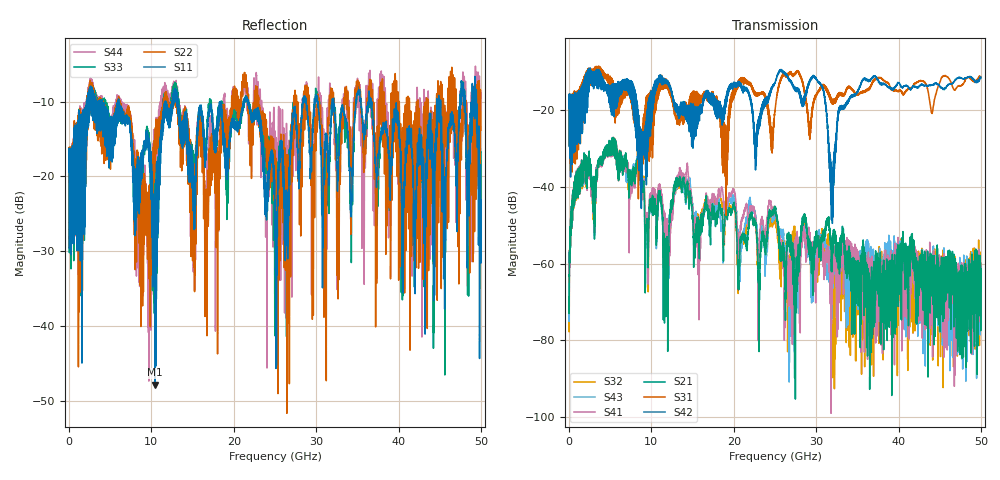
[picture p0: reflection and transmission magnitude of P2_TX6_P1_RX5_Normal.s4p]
!Keysight Technologies,N5225B,MY57041031,A.13.20.10
!Date: Friday, May 31, 2019 11:21:51
!Correction: S11(Full 4 Port(1,2,3,4))
!S12(Full 4 Port(1,2,3,4))
!S13(Full 4 Port(1,2,3,4))
!S14(Full 4 Port(1,2,3,4))
!S21(Full 4 Port(1,2,3,4))
!S22(Full 4 Port(1,2,3,4))
!S23(Full 4 Port(1,2,3,4))
!S24(Full 4 Port(1,2,3,4))
!S31(Full 4 Port(1,2,3,4))
!S32(Full 4 Port(1,2,3,4))
!S33(Full 4 Port(1,2,3,4))
!S34(Full 4 Port(1,2,3,4))
!S41(Full 4 Port(1,2,3,4))
!S42(Full 4 Port(1,2,3,4))
!S43(Full 4 Port(1,2,3,4))
!S44(Full 4 Port(1,2,3,4))
!S4P File: Measurements: <S11,S12,S13,S14>,
!<S21,S22,S23,S24>,
!<S31,S32,S33,S34>,
!<S41,S42,S43,S44>:
# Hz S  dB  R 50.0
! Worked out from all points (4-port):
!   5000 points, 10 MHz to 50 GHz, reference 50 ohm
!   strongest paths, dB at 10 MHz, 12.51 GHz, 25.01 GHz, 37.51 GHz, 50 GHz:
!     S42: -19.4, -15.5, -12.9, -12.0, -11.3
!     S31: -19.3, -16.8, -20.0, -11.6, -11.4
!     S21: -68.7, -45.3, -45.4, -64.1, -66.3
!     S41: -56.9, -48.0, -46.6, -71.4, -65.6
!     S43: -56.7, -47.7, -47.7, -59.4, -63.1
!     S32: -63.0, -47.4, -48.1, -58.6, -72.7
!   lowest |S11| = -47.8 dB at 10.41 GHz (marker M1), VSWR 1.01, Z = 50.1 - j0.405 ohm
!   |S11| at or under -10 dB: 13.21 GHz to 21.18 GHz (7.966 GHz wide, 46.3 % of centre); 21.74 GHz to 28.38 GHz (6.638 GHz wide, 26.5 % of centre); 36.67 GHz to 44.63 GHz (7.961 GHz wide, 19.6 % of centre)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
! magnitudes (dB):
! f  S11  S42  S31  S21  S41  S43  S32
! 10 MHz  -19.4  -19.4  -19.3  -68.7  -56.9  -56.7  -63.0
! 5.11 GHz  -13.9  -16.3  -13.0  -28.5  -28.4  -28.1  -28.4
! 10.41 GHz  -47.8  -14.2  -14.8  -43.9  -41.5  -43.3  -43.0
! 29.79 GHz  -9.8  -11.1  -16.8  -54.6  -62.1  -58.8  -56.3
! 31.9 GHz  -11.8  -38.5  -17.7  -59.4  -59.2  -64.4  -62.4
! 35.77 GHz  -14.2  -11.7  -15.0  -55.8  -66.4  -66.1  -57.7
! 50 GHz  -23.1  -11.3  -11.4  -66.3  -65.6  -63.1  -72.7
